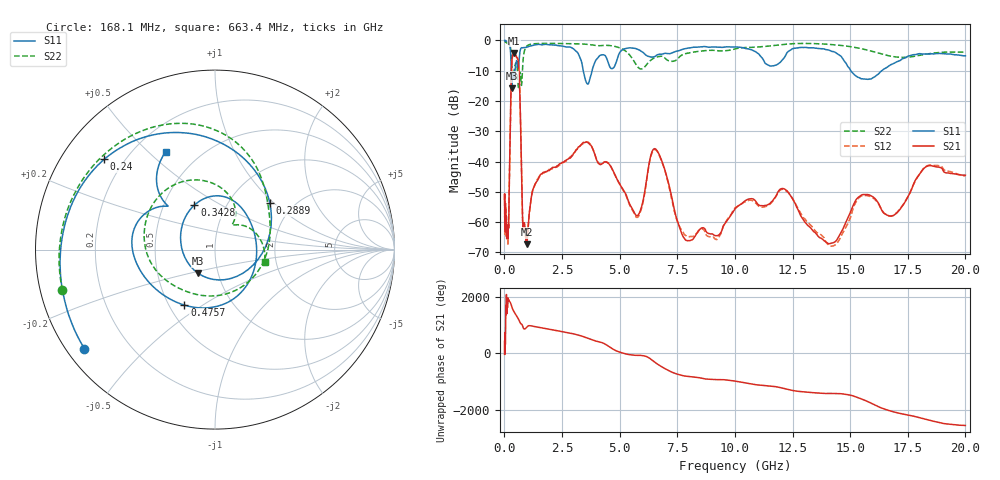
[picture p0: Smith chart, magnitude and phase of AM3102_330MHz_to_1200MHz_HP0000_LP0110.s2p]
! Date/Time: Tue, Sep 11, 2018 5:08 PM
! Network Analyzer: Agilent Technologies E8362B Rev: A.07.50.63
! Sweep from 0.010 to 20.000 GHz, 1601 Points, Sweep Type: LOG
! Power Supply: 4.950 V, 0.001 A
# Hz S DB R 50
!freq MagS11 AngS11 MagS21 AngS21 MagS12 AngS12 MagS22 AngS22
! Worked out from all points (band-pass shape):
!   1601 points, 10 MHz to 20 GHz, reference 50 ohm
!   highest |S21| = -4.13 dB at 416.5 MHz (marker M1); lowest = -67.3 dB at 974.7 MHz (marker M2)
!   |S21| within 3 dB of the highest: 322.2 MHz to 606.8 MHz (284.6 MHz wide, 61.3 % of centre)
!   lowest |S11| = -15.8 dB at 316.2 MHz (marker M3), VSWR 1.39, Z = 40.1 - j10.8 ohm
!   |S11| at or under -10 dB: 294.7 MHz to 456.6 MHz (161.9 MHz wide, 43.1 % of centre); 3.422 GHz to 3.804 GHz (381.5 MHz wide, 10.6 % of centre); 15.03 GHz to 16.38 GHz (1.348 GHz wide, 8.58 % of centre)
!   |S22| runs from -15.6 to -0.2 dB; largest |S21 - S12| = 0.01
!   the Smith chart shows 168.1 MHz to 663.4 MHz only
!   S11 on the Smith chart (normalised r, x): 168.1 MHz: 0.05, -0.34; 240 MHz: 0.13, +0.35; 288.9 MHz: 1.52, +0.95; 342.8 MHz: 0.71, +0.38; 475.7 MHz: 0.60, -0.42; 663.4 MHz: 0.33, +0.57
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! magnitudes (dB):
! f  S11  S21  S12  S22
! 10 MHz  0.0  -52.4  -52.6  -0.2
! 35.55 MHz  0.0  -60.0  -63.8  -0.4
! 126.4 MHz  -0.4  -63.6  -62.8  -0.9
! 168.1 MHz  -0.8  -62.0  -63.2  -1.1
! 240 MHz  -2.0  -35.7  -35.8  -1.8
! 288.9 MHz  -7.9  -14.7  -14.8  -3.9
! 316.2 MHz  -15.8  -7.9  -7.9  -7.3
! 342.8 MHz  -11.3  -5.6  -5.7  -10.3
! 416.5 MHz  -12.5  -4.1  -4.2  -10.4
! 447.2 MHz  -10.5  -4.3  -4.3  -8.7
! 475.7 MHz  -9.0  -4.6  -4.6  -7.8
! 663.4 MHz  -4.3  -15.8  -15.9  -10.9
! 798.4 MHz  -2.4  -60.5  -61.3  -7.8
! 974.7 MHz  -2.2  -67.3  -66.5  -1.9
! 1.59 GHz  -1.4  -44.1  -44.3  -1.0
! 3.599 GHz  -14.4  -33.7  -33.5  -1.3
! 5.652 GHz  -2.6  -57.1  -57.4  -7.2
! 6.58 GHz  -5.0  -36.0  -36.3  -5.6
! 7.92 GHz  -2.6  -66.1  -64.7  -4.3
! 12.09 GHz  -6.2  -48.9  -49.2  -1.4
! 14.14 GHz  -3.4  -67.1  -68.0  -1.3
! 20 GHz  -5.1  -44.5  -44.8  -3.9
